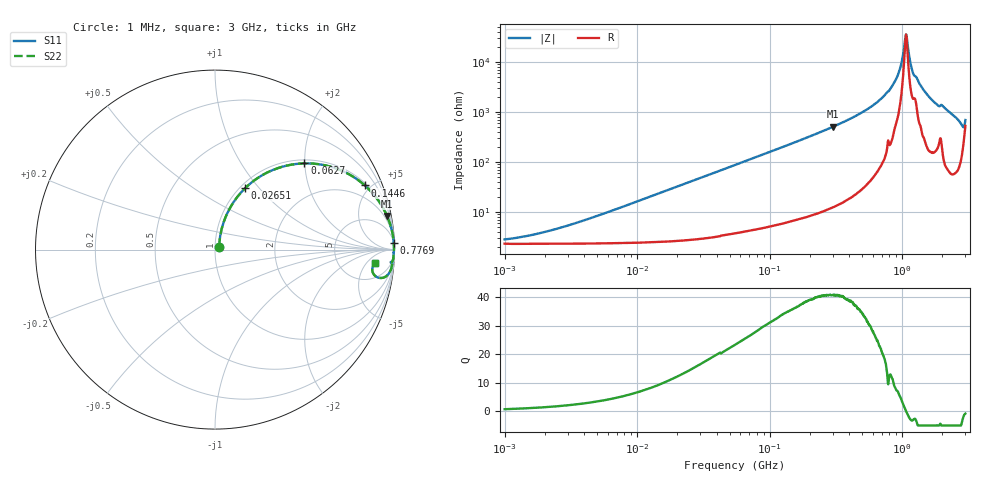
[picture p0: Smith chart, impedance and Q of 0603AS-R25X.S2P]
!s-Parameter Generated by FASTRON Sdn. Bhd.
!FASTRON P/N : 0603AS-R25X
!Keysight Technologies: E4991B_MY54100416_A.01.15
!Date created: Tue Oct 17 15:04:22 2023
!Version  : Rev01 Tue Oct 17 15:04:22 2023
!Data & Calibration Information:
!Freq	S11	S21	S12	S22
!PortZ  Port1:50+j0  Port2:50+j0
!When reading reference impedance value at option line is always used.
! Remarks : This data is being provided solely for informational purposes.
# Hz S dB R 50
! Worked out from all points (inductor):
!   1601 points, 1 MHz to 3 GHz, reference 50 ohm
!   read as one part in series: L = 256 nH near 4.376 MHz
!   highest Q = 40.8 at 301.7 MHz (marker M1), where L = 268 nH
!   self-resonance near 1.07 GHz
!   S11 on the Smith chart (normalised r, x): 1 MHz: 1.05, +0.03; 26.51 MHz: 1.06, +0.85; 62.7 MHz: 1.08, +1.99; 144.6 MHz: 1.13, +4.61; 776.9 MHz: 6, +51; 3 GHz: 12, -9
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1000000  -31.14 34.0  -0.20 -0.9  -0.20 -0.9  -31.14 34.0
3804036  -23.88 65.7  -0.22 -3.4  -0.22 -3.4  -23.88 65.7
1.447069e7  -13.08 71.1  -0.43 -12.7  -0.43 -12.7  -13.08 71.1
2.651225e7  -8.37 63.8  -0.92 -22.4  -0.92 -22.4  -8.37 63.8
5.477226e7  -3.83 47.5  -2.63 -40.0  -2.63 -40.0  -3.83 47.5
6.26956e7  -3.20 43.9  -3.17 -43.8  -3.17 -43.8  -3.20 43.9
1.445978e8  -0.84 23.2  -8.10 -65.2  -8.10 -65.2  -0.84 23.2
2.083556e8  -0.42 16.4  -11.00 -72.2  -11.00 -72.2  -0.42 16.4
3.017325e8  -0.20 11.1  -14.34 -77.5  -14.34 -77.5  -0.20 11.1
5.445776e8  -0.06 5.0  -21.14 -83.1  -21.14 -83.1  -0.06 5.0
7.768855e8  -0.04 2.2  -28.17 -82.5  -28.17 -82.5  -0.04 2.2
7.925923e8  -0.04 2.2  -28.41 -82.6  -28.41 -82.6  -0.04 2.2
9.349007e8  -0.02 1.0  -35.27 -80.3  -35.27 -80.3  -0.02 1.0
9.878038e8  -0.02 0.6  -39.59 -75.2  -39.59 -75.2  -0.02 0.6
1.0437e9  -0.02 0.2  -47.50 -49.8  -47.50 -49.8  -0.02 0.2
1.070143e9  -0.02 0.0  -51.04 -1.8  -51.04 -1.8  -0.02 0.0
1.097256e9  -0.03 -0.2  -47.41 47.0  -47.41 47.0  -0.03 -0.2
1.159346e9  -0.03 -0.6  -39.15 71.1  -39.15 71.1  -0.03 -0.6
1.206698e9  -0.04 -0.9  -35.64 71.3  -35.64 71.3  -0.04 -0.9
1.488926e9  -0.04 -2.2  -28.09 82.1  -28.09 82.1  -0.04 -2.2
2.811057e9  -0.47 -9.6  -15.36 67.2  -15.36 67.2  -0.47 -9.6
3e9  -0.94 -4.8  -17.74 35.3  -17.74 35.3  -0.94 -4.8
